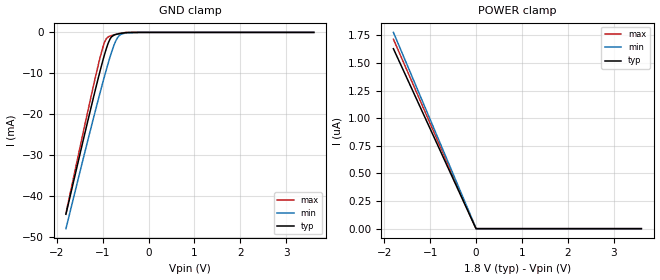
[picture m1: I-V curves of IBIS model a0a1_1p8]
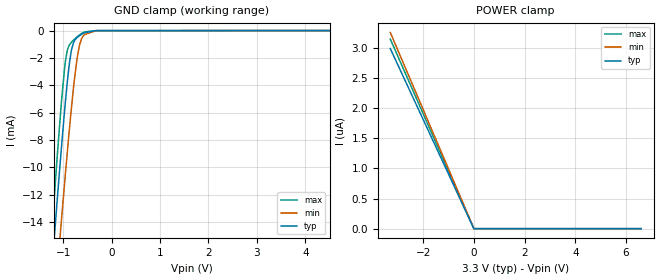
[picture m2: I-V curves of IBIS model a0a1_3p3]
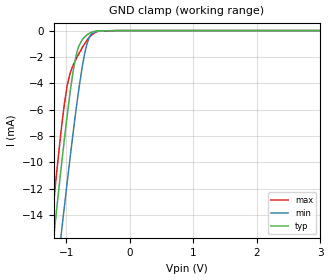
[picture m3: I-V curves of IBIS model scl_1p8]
|Texas Instruments Incorporated
|4.5V to 17V Input, 12A/9A/7A/5A Output, Synchronous Step-Down Voltage
|Marketing part#   Digital Voltage Range   Package-type   #pins
|TPS56520PWP   4.5V-17V   HTSSOP   20
|TPS56720PWP   4.5V-17V   HTSSOP   20
|TPS56920PWP   4.5V-17V   HTSSOP   20
|TPS56C20PWP   4.5V-17V   HTSSOP   20
|TPS56520PWP   4.5V-17V   HTSSOP   24
[IBIS Ver]   4.1
[File name]   tps56520.ibs
[File Rev]   1.0
[Date]   9/29/2016
[Source]
| Texas Instruments Incorporated.
| Analog-eLab Design Center, HPA
| 12500 TI Blvd
| Dallas, TX -75243
[Notes]   Revision History:
| Rev 1.0: 9/29/2016
| - Initial version of the model
| - Model generated from simulations in SPECTRE
| - Model matched to SPICE simulation
| - C_comp although listed in numerical order of value are
|   obtained from varying PVT conditions. For PVT conditions for
|   each specific value refer the buffer description under
|   respective [Model]. IBIS model user is responsible for using
|   appropriate C_comp to simulate for Signal Integrity.
|*EXCEPTION:   *
|* -For model a0a1_*,there will be leakage in ground clamp IV table   *
|*  because of Resistor R0 connected to pad.   *
|* -For model en_*,there will be leakage in power and ground clamp   *
|*  IV tables because of transistors(MN9, MN8) connected to pad.   *
|* -For model sda_*, pulldown IV table does not pass through 0 because   *
|*  of driver transistor MN5 connected to pad.   *
[Disclaimer]
| This model is designed as an aid for customers of Texas Instruments.
| TI and its licensors and suppliers make no warranties, either expressed
| or implied, with respect to this  model, including the warranties of
| merchantability or fitness for a particular purpose. The model is
| provided solely on an "as is" basis. The entire risk as to its quality
| and performance is with the customer.
[Copyright]
(C) Copyright 2016 Texas Instruments Incorporated.All rights reserved.
|   TPS56520PWP
[Component]   TPS56520PWP
[Manufacturer]   TI
[Package]   |20 HTSSOP  -  PWP package
|   typ   min   max
R_pkg   0.2   0.16   0.24
L_pkg   1.5nH   1.2nH   1.8nH
C_pkg   0.4pF   0.32pF   0.48pF
[Pin]  signal_name   model_name   R_pin   L_pin   C_pin
1   EN   en   NA   NA   NA
2   SDA   sda   NA   NA   NA
3   SCL   scl   NA   NA   NA
4   A1   a0a1   NA   NA   NA
5   A0   a0a1   NA   NA   NA
6   VIN   power   NA   NA   NA
7   PVIN   power   NA   NA   NA
8   PVIN   power   NA   NA   NA
9   PGND   gnd   NA   NA   NA
10   PGND   gnd   NA   NA   NA
11   SW   nc   NA   NA   NA
12   SW   nc   NA   NA   NA
13   SW   nc   NA   NA   NA
14   VBST   power   NA   NA   NA
15   PGOOD   nc   NA   NA   NA
16   VREG5   power   NA   NA   NA
17   GND   gnd   NA   NA   NA
18   SS   nc   NA   NA   NA
19   VOUT   nc   NA   NA   NA
20   VFB   nc   NA   NA   NA
|   Model Selectors
[Model Selector] a0a1
a0a1_1p8  1.8V  digital Input
a0a1_3p3  3.3V  digital Input
[Model Selector] scl
scl_1p8   1.8V  digital Input
scl_3p3   3.3V  digital Input
[Model Selector] en
en_1p8   1.8V  digital Input
en_3p3   3.3V  digital Input
[Model Selector] sda
sda_1p8   1.8V  digital Input
sda_3p3   3.3V  digital Input
| Models and submodels in the file (8): a0a1_1p8 (Input), a0a1_3p3 (Input), scl_1p8 (Input), scl_3p3 (Input), en_1p8 (Input), en_3p3 (Input), sda_1p8 (I/O_open_drain), sda_3p3 (I/O_open_drain)
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|   a0a1_1p8 Model
[Model]   a0a1_1p8
Model_type   Input
Vinl = 0.6
Vinh = 1.26
|   typ   min   max
|   (nom PVT)   (fast PVT)   (slow PVT)
C_comp   4.568e-13   4.568e-13   4.630e-13
| Where nom  PVT is Nominal Process, 1.8V, 27C
|   Fast PVT is Strong Process,  1.9V, -40C
|   Slow PVT is Weak Process,   1.7V, 125C
[Voltage Range]   1.8   1.7   1.9
|Junction Temperature
[Temperature Range]   27   125   -40
[Power Clamp Reference]   1.8   1.7   1.9
[GND Clamp Reference]   0   0   0
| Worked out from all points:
|   GND clamp passes 1 mA (typ) near -0.80 V on its own axis
[GND Clamp]
|   Voltage   I(typ)   I(min)   I(max)
-1.8V     -44.52mA   -48.04mA   -44.28mA
-1.435V   -26.96mA   -31.45mA   -25.06mA
-1.192V   -15.55mA   -20.63mA   -12.63mA
-1.089V   -10.91mA   -16.17mA   -7.675mA
-994.4mV  -6.841mA   -12.16mA   -3.608mA
-920.3mV  -3.98mA    -9.135mA   -1.549mA
-837mV    -1.587mA   -5.941mA   -886.1uA
-723.6mV  -545.4uA   -2.32mA    -495uA
-638.9mV  -316.4uA   -775.8uA   -260.6uA
-509.9mV  -84.15uA   -170.7uA   -38.8uA
-180mV    -1.805uA   -2.266uA   -1.983uA
3.6V      0A         0A         0A
[POWER Clamp]
|   Voltage   I(typ)   I(min)   I(max)
-1.8V     1.629uA    1.777uA    1.715uA
-21.6mV   17.99nA    24.01nA    18.81nA
0V        0A         0A         0A
3.6V      0A         0A         0A
|   a0a1_3p3 Model
[Model]   a0a1_3p3
Model_type   Input
Vinl = 0.6
Vinh = 1.8
|   typ   min   max
|   (nom PVT)   (fast PVT)   (slow PVT)
C_comp   4.568e-13   4.568e-13   4.630e-13
| Where nom  PVT is Nominal Process, 3.3V, 27C
|   Fast PVT is Strong Process,  3.6V, -40C
|   Slow PVT is Weak Process,   3V, 125C
[Voltage Range]   3.3   3   3.6
|Junction Temperature
[Temperature Range]   27   125   -40
[Power Clamp Reference]   3.3   3   3.6
[GND Clamp Reference]   0   0   0
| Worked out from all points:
|   GND clamp passes 1 mA (typ) near -0.80 V on its own axis
[GND Clamp]
|   Voltage   I(typ)   I(min)   I(max)
-3.3V     -118.2mA   -117.6mA   -124.7mA
-1.244V   -17.88mA   -22.86mA   -15.15mA
-1.198V   -15.75mA   -20.83mA   -12.84mA
-1.118V   -12.14mA   -17.37mA   -8.96mA
-1.076V   -10.25mA   -15.54mA   -6.971mA
-1.038V   -8.609mA   -13.93mA   -5.296mA
-951mV    -5.057mA   -10.32mA   -2.16mA
-831.6mV  -1.455mA   -5.698mA   -858uA
-714mV    -509.9uA   -2.051mA   -461.8uA
-663.3mV  -371.4uA   -1.069mA   -319.3uA
-564mV    -163.2uA   -299.8uA   -103.9uA
6.6V      0A         0A         0A
[POWER Clamp]
|   Voltage   I(typ)   I(min)   I(max)
-3.3V     2.987uA    3.255uA    3.144uA
-27.6mV   22.08nA    29.14nA    22.92nA
0V        0A         0A         0A
6.6V      0A         0A         0A
|   scl_1p8 Model
[Model]   scl_1p8
Model_type   Input
Vinl = 0.6
Vinh = 1.26
|   typ   min   max
|   (nom PVT)   (fast PVT)   (slow PVT)
C_comp   7.305e-13   6.913e-13   7.721e-13
| Where nom  PVT is Nominal Process, 1.8V, 27C
|   Fast PVT is Strong Process,  1.9V, -40C
|   Slow PVT is Weak Process,   1.7V, 125C
[Voltage Range]   1.8   1.7   1.9
|Junction Temperature
[Temperature Range]   27   125   -40
[Power Clamp Reference]   1.8   1.7   1.9
[GND Clamp Reference]   0   0   0
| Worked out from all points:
|   GND clamp passes 1 mA (typ) near -0.78 V on its own axis
[GND Clamp]
|   Voltage   I(typ)   I(min)   I(max)
-1.8V     -44.34mA   -47.76mA   -44.18mA
-1.385V   -24.43mA   -28.94mA   -22.45mA
-1.22V    -16.73mA   -21.62mA   -14.14mA
-1.154V   -13.69mA   -18.7mA    -10.92mA
-1.079V   -10.38mA   -15.49mA   -7.547mA
-985.7mV  -6.46mA    -11.55mA   -4.197mA
-874.7mV  -2.616mA   -7.111mA   -2.453mA
-814mV    -1.353mA   -4.879mA   -1.869mA
-741.7mV  -657.5uA   -2.566mA   -1.247mA
-640.6mV  -214.7uA   -551.9uA   -535.7uA
-490.9mV  -20.28uA   -29.73uA   -44.92uA
3.6V      0A         0A         0A
[POWER Clamp]
|   Voltage   I(typ)   I(min)   I(max)
-1.8V     0A         0A         0A
0V        0A         0A         0A
3.6V      0A         0A         0A
